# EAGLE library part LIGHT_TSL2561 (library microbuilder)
TSL2561 Light-To-Digital Sensor Mouser Part Numbers: CS (obsolete): 856-TSL2561CS DFN (cheapest): 856-TSL2561FN
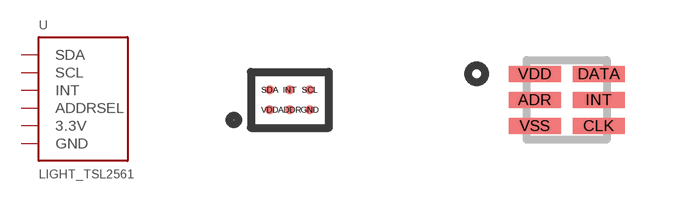
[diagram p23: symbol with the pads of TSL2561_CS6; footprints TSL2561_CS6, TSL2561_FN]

Designator prefix U

## LIGHT_TSL2561CS  [TSL2561_CS6]
ADDR  ADDRSEL
GND  GND
INT  INT
SCL  SCL
SDA  SDA
VDD  3.3V

## LIGHT_TSL2561  [TSL2561_FN]
ADR  ADDRSEL
CLK  SCL
DATA  SDA
INT  INT
VDD  3.3V
VSS  GND

## Footprint TSL2561_CS6 (pad centres in mm)
6 Lead Chipscale 0.21mm pads, 0.5mm pitch
smd 0.21 x 0.21: ADDR 0,-0.25; GND 0.5,-0.25; INT 0,0.25; SCL 0.5,0.25; SDA -0.5,0.25; VDD -0.5,-0.25

## Footprint TSL2561_FN (pad centres in mm)
2.0x2.0mm DFN (0.65mm pitch)
smd 1.3 x 0.4: ADR -0.8,0; CLK 0.8,-0.65; DATA 0.8,0.65; INT 0.8,0; VDD -0.8,0.65; VSS -0.8,-0.65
